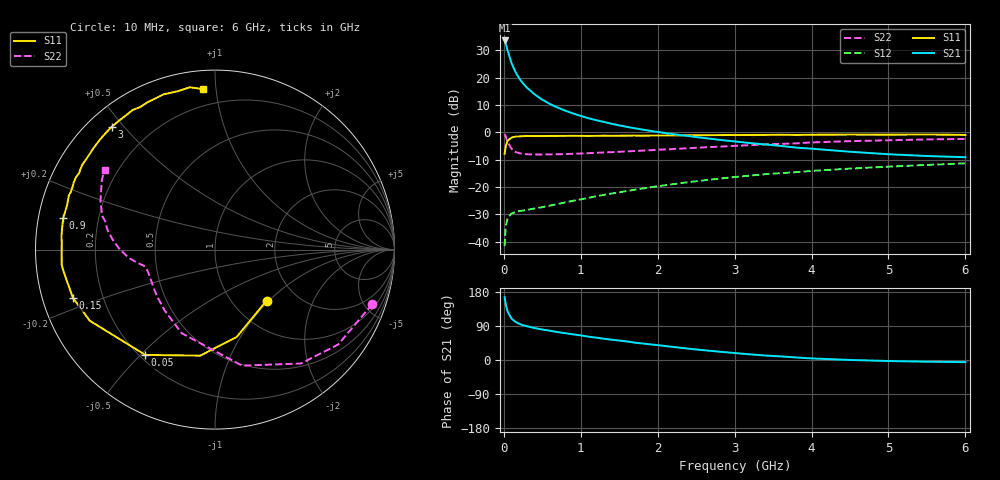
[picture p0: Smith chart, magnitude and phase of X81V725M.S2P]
! SIEMENS Small Signal Semiconductors
! BFP136W
! Si NPN RF Bipolar Junction Transistor in SOT343
! VCE = 1.75 V  IC = 25 mA
! Common Emitter S-Parameters:  September  1994
# GHz  S  MA  R  50
!  f  S11  S21  S12  S22
! GHz  MAG  ANG  MAG  ANG  MAG  ANG  MAG  ANG
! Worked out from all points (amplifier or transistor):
!   40 points, 10 MHz to 6 GHz, reference 50 ohm
!   highest |S21| = 33.6 dB at 10 MHz (marker M1)
!   |S21| within 3 dB of that: start of sweep to 42.88 MHz
!   unconditionally stable (mu >= 1): 789.5 MHz to 2.781 GHz
!   at 200 MHz: K = 0.39, MSG = 24.2 dB, |S12| = -28.8 dB
!   at 1.5 GHz: K = 1.16, MAG = 9.8 dB, |S12| = -21.9 dB
!   at 6 GHz: K = 0.99, MSG = 1.1 dB, |S12| = -11.3 dB
!   S11 on the Smith chart (normalised r, x): 10 MHz: 1.42, -0.97; 50 MHz: 0.22, -0.52; 150 MHz: 0.09, -0.16; 900 MHz: 0.07, +0.10; 3 GHz: 0.07, +0.46; 6 GHz: 0.10, +0.92
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0.01  0.4042 -44.6  47.84 165.9  0.0083 75.6  0.9278 -19.1
0.02  0.5013 -76.0  43.84 152.9  0.0151 64.0  0.8664 -37.6
0.03  0.5965 -97.9  39.77 142.5  0.0207 56.3  0.7948 -53.0
0.05  0.7036 -123.5  31 127.3  0.0273 41.6  0.6637 -76.9
0.1  0.8024 -150.4  18.46 109.2  0.0329 29.5  0.5011 -111.8
0.15  0.8357 -161.2  12.8 100.7  0.0348 26.2  0.4398 -129.6
0.2  0.8421 -167.3  9.682 95.5  0.0364 25.6  0.4163 -140.1
0.25  0.8524 -171.7  7.839 91.9  0.0372 26.6  0.4048 -147.0
0.3  0.8583 -174.4  6.565 89.1  0.0382 27.5  0.3976 -151.6
0.4  0.8547 -179.2  4.946 84.3  0.0405 30.8  0.3936 -157.6
0.5  0.8545 177.4  3.947 80.4  0.0429 34.1  0.3931 -161.2
0.6  0.8586 175.1  3.293 77.2  0.0458 37.0  0.3952 -163.4
0.7  0.8602 171.9  2.838 73.6  0.0489 40.1  0.3977 -164.8
0.9  0.8636 168.3  2.215 67.7  0.0561 44.2  0.4052 -167.0
1.1  0.8599 163.6  1.811 61.5  0.0635 47.7  0.4165 -168.3
1.5  0.8662 156.6  1.339 51.2  0.0803 51.7  0.4407 -170.7
2.2  0.8771 144.0  0.927 34.5  0.1129 52.1  0.4953 -176.1
3  0.8937 130.1  0.683 18.4  0.1524 47.8  0.5657 175.5
3.2  0.8955 126.7  0.637 14.9  0.1618 46.1  0.5828 173.0
4.5  0.9111 108.2  0.442 0.1  0.2174 34.8  0.6908 157.5
5.5  0.915 98.8  0.369 -4.5  0.2539 26.5  0.7414 148.2
6  0.8962 94.2  0.351 -5.6  0.2711 22.0  0.7587 144.2
